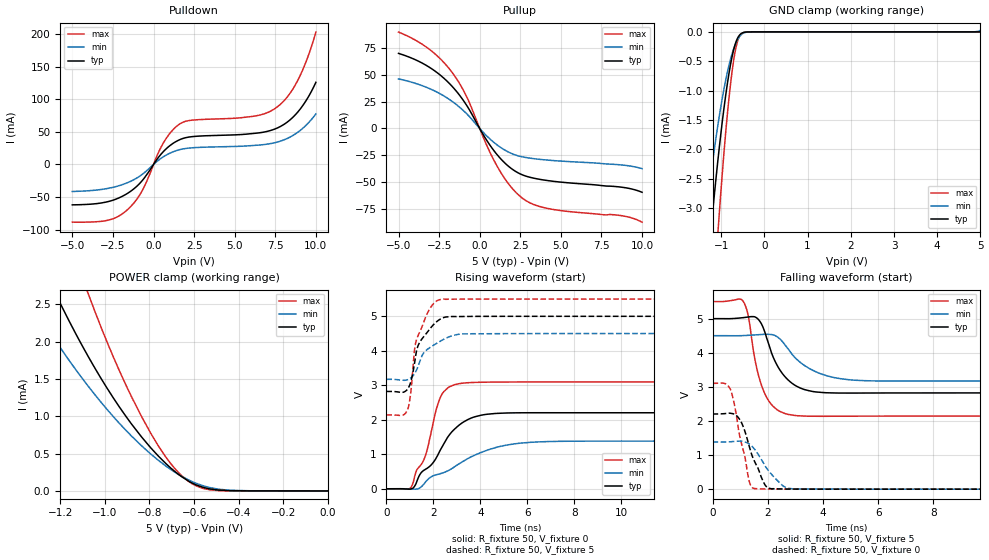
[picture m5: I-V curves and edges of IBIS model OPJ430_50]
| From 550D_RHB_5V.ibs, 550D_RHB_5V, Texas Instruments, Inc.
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[Model]   OPJ430_50
Model_type  3-state
Enable   Active-Low
Vref =   2.5
Rref =   50
Cref =   15p
Vmeas =   2.5
| variable   typ   min   max
C_comp   0.49pF   0.45pF   0.53pF
| C_pullup   1.53pF   0.39pF   2.17pF
| C_pulldown   1.30pF   0.59pF   2.02pF
| C_tri-state   0.49pF   0.45pF   0.53pF
[Temperature Range]   40   125   -40
| Ambient temperature   25   110   -40
[Voltage range]   5   4.5   5.5
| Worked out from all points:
|   slope of the pulldown table from 0 to 0.75 V, typ, clamps not added: 32.2 ohm
|   slope of the pullup table from 0 to 0.75 V, typ, clamps not added: 41.5 ohm
|   GND clamp passes 1 mA (typ) near -0.88 V on its own axis
|   POWER clamp passes 1 mA (typ) near -0.91 V on its own axis
|   rising waveform, R_fixture 50, V_fixture 0: 20-80 % time 1.5ns typ, 2.46ns min, 829ps max; typ from 0 V to 2.2 V
|   falling waveform, R_fixture 50, V_fixture 5: 20-80 % time 760ps typ, 1.13ns min, 538ps max; typ from 5 V to 2.82 V
|   rising waveform, R_fixture 50, V_fixture 5: 20-80 % time 677ps typ, 905ps min, 547ps max; typ from 2.82 V to 5 V
|   falling waveform, R_fixture 50, V_fixture 0: 20-80 % time 584ps typ, 739ps min, 449ps max; typ from 2.2 V to 0 V
[GND Clamp]
| OPJ430_50
|   Voltage   I(typ)   I(min)   I(max)
-5V       -50.89mA   -38mA      -68.64mA
-1.39V    -4.679mA   -3.339mA   -7.149mA
-1.365V   -4.459mA   -3.183mA   -6.826mA
-1.225V   -3.294mA   -2.362mA   -5.098mA
-1.075V   -2.184mA   -1.584mA   -3.42mA
-1.04V    -1.948mA   -1.42mA    -3.059mA
-950mV    -1.387mA   -1.032mA   -2.192mA
-870mV    -951.3uA   -733.5uA   -1.509mA
-745mV    -413.9uA   -366.2uA   -662.7uA
-630mV    -121.8uA   -145.9uA   -183.2uA
-500mV    -14.79uA   -27.21uA   -15.48uA
5V        149.5pA    27.58uA    104.4pA
[POWER Clamp]
| OPJ430_50
|   Voltage   I(typ)   I(min)   I(max)
-5V       53.25mA    39.29mA    70.31mA
-1.37V    3.631mA    2.724mA    5.412mA
-1.34V    3.422mA    2.574mA    5.098mA
-1.22V    2.637mA    2.01mA     3.914mA
-1.075V   1.804mA    1.405mA    2.647mA
-935mV    1.126mA    906.2uA    1.612mA
-835mV    721.6uA    603.7uA    994.1uA
-725mV    362.2uA    330uA      446.7uA
-625mV    131.9uA    147.4uA    128.2uA
-560mV    48.15uA    69.52uA    33.43uA
-490mV    11.07uA    23.1uA     4.422uA
-84.4fV   149.5pA    523.8pA    122.1pA
[Pulldown]
| OPJ430_50
|   Voltage   I(typ)   I(min)   I(max)
-5V       -61.89mA   -41.4mA    -88.4mA
-2.815V   -57.01mA   -36.69mA   -85.54mA
-1.595V   -44.17mA   -27.83mA   -69.1mA
-685mV    -24.41mA   -14.96mA   -39.62mA
685mV     21.77mA    13.02mA    36.26mA
1.68V     38.72mA    23.14mA    63.14mA
6.295V    47.91mA    29.41mA    74.47mA
7.65V     56.24mA    34.57mA    88.8mA
8.3V      66.21mA    40.68mA    105.5mA
8.9V      80.88mA    49.68mA    129.8mA
9.46V     100.5mA    61.8mA     161.9mA
10V       126mA      77.5mA     203mA
[Pullup]
| OPJ430_50
|   Voltage   I(typ)   I(min)   I(max)
-5V       69.87mA    46.14mA    89.69mA
-3.13V    57.25mA    37.38mA    74.02mA
-1.7V     39.22mA    25.25mA    52.2mA
-795mV    21.32mA    13.58mA    29.33mA
360mV     -9.264mA   -5.829mA   -13.14mA
1.06V     -24.13mA   -15.16mA   -34.71mA
1.825V    -35.8mA    -22.32mA   -52.46mA
2.6V      -42.96mA   -26.31mA   -64.49mA
3.275V    -46.05mA   -27.96mA   -70.42mA
4.195V    -48.49mA   -29.43mA   -74.43mA
8.69V     -54.53mA   -33.87mA   -81.03mA
10V       -59.36mA   -37.37mA   -87.19mA
[Ramp]
| OPJ430_50
| variable   typ   min   max
dV/dt_r   1.33/1.51E-09   0.84/2.49E-09   1.86/8.45E-10
dV/dt_f   1.34/7.81E-10   0.82/1.16E-09   2.06/5.49E-10
R_load = 50
[Rising Waveform]
| OPJ430_50
R_fixture =   50
C_fixture =   0
L_fixture =   0
V_fixture =   0
V_fixture_min = 0
V_fixture_max = 0
|   Time   V(typ)   V(min)   V(max)
0s        -408nV     -5.152uV   343.7nV
1.045ns   -5.02mV    -6.859mV   35.51mV
1.285ns   189mV      -8.604mV   527.9mV
1.675ns   568.8mV    203.5mV    983.6mV
2.07ns    834.8mV    393.5mV    2.161V
2.315ns   1.145V     441.5mV    2.673V
3.125ns   1.861V     736.2mV    3.05V
4.175ns   2.151V     1.089V     3.09V
6.41ns    2.204V     1.357V     3.097V
24.99ns   2.204V     1.382V     3.099V
[Falling Waveform]
| OPJ430_50
R_fixture =   50
C_fixture =   0
L_fixture =   0
V_fixture =   5
V_fixture_min = 4.5
V_fixture_max = 5.5
|   Time   V(typ)   V(min)   V(max)
0s        5V         4.5V       5.5V
1.11ns    5.029V     4.503V     5.508V
1.295ns   5.048V     4.511V     5.08V
1.61ns    5.016V     4.526V     3.522V
1.875ns   4.653V     4.54V      2.835V
2.34ns    3.635V     4.469V     2.33V
2.905ns   3.091V     3.932V     2.17V
3.965ns   2.835V     3.371V     2.137V
5.505ns   2.819V     3.181V     2.141V
24.99ns   2.822V     3.173V     2.142V
[Rising Waveform]
| OPJ430_50
R_fixture =   50
C_fixture =   0
L_fixture =   0
V_fixture =   5
V_fixture_min = 4.5
V_fixture_max = 5.5
|   Time   V(typ)   V(min)   V(max)
0s        2.822V     3.173V     2.142V
880ps     2.871V     3.157V     2.262V
1.025ns   3.067V     3.205V     2.711V
1.2ns     3.639V     3.339V     4.024V
1.275ns   3.961V     3.429V     4.299V
1.555ns   4.38V      3.904V     4.764V
1.855ns   4.636V     4.094V     5.225V
2.34ns    4.936V     4.295V     5.494V
3.67ns    4.997V     4.495V     5.5V
24.99ns   5V         4.5V       5.5V
[Falling Waveform]
| OPJ430_50
R_fixture =   50
C_fixture =   0
L_fixture =   0
V_fixture =   0
V_fixture_min = 0
V_fixture_max = 0
|   Time   V(typ)   V(min)   V(max)
0s        2.204V     1.382V     3.101V
650ps     2.225V     1.39V      2.925V
785ps     2.202V     1.4V       2.512V
1.03ns    1.985V     1.409V     1.399V
1.325ns   1.275V     1.326V     250.6mV
1.52ns    820.3mV    1.174V     16.68mV
1.985ns   52.96mV    588.1mV    4.771mV
2.545ns   6.035mV    101.9mV    860.6uV
2.94ns    3.176mV    6.524mV    144.6uV
24.99ns   330.2nV    227.7nV    101.7nV
